(* Logix 5000 AddOnInstructionDefinition export Banner_IOL_Analog_Converter_Param_v4; software revision 33.00; part 2 of 2 *)
(* tags used below, declared in another part *)
   Converter : Banner_Analog_Converter_v4;
   Port_Data : Banner_IOL_Port_v4;
   Port : DINT;
   Type : DINT;   // 0 for S15C U/I models. 1 for R45C U/I models. 2 for R45C UU/II double analog models.
   Local_Control : DINT;
   Command_Being_Processed : BOOL;
   Index_Write_Inprocess : INT;
   Index_Write_Control : INT;
   Update_Archive : BOOL;
   Inprocess_Index : DINT;
   Index : DINT;
   Index2 : DINT;
   Index3 : DINT;
(* Banner_IOL_Analog_Converter_Param_v4, continued *)

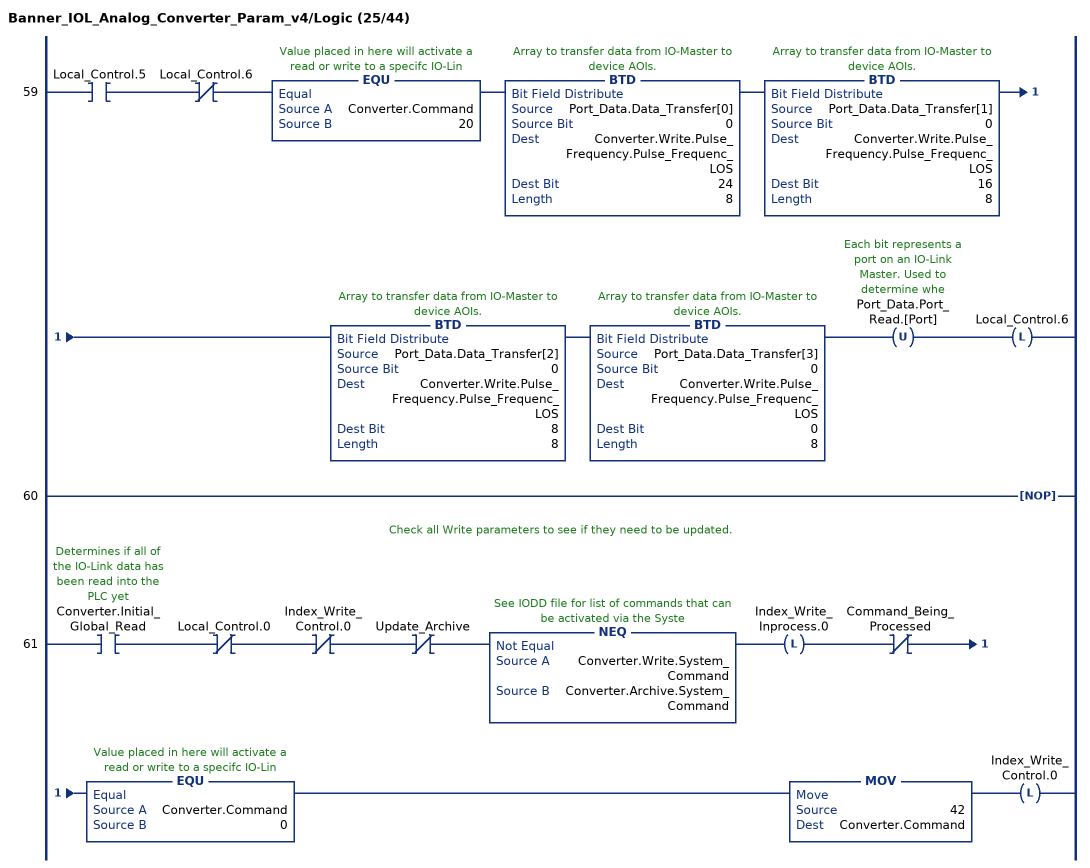
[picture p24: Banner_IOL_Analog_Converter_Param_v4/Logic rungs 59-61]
   59: XIC(Local_Control.5)XIO(Local_Control.6)EQU(Converter.Command,20)BTD(Port_Data.Data_Transfer[0],0,Converter.Write.Pulse_Frequency.Pulse_Frequenc_LOS,24,8)BTD(Port_Data.Data_Transfer[1],0,Converter.Write.Pulse_Frequency.Pulse_Frequenc_LOS,16,8)BTD(Port_Data.Data_Transfer[2],0,Converter.Write.Pulse_Frequency.Pulse_Frequenc_LOS,8,8)BTD(Port_Data.Data_Transfer[3],0,Converter.Write.Pulse_Frequency.Pulse_Frequenc_LOS,0,8)OTU(Port_Data.Port_Read.[Port])OTL(Local_Control.6);
   60: NOP();
   // Check all Write parameters to see if they need to be updated.
   61: XIC(Converter.Initial_Global_Read)XIO(Local_Control.0)XIO(Index_Write_Control.0)XIO(Update_Archive)NEQ(Converter.Write.System_Command,Converter.Archive.System_Command)OTL(Index_Write_Inprocess.0)XIO(Command_Being_Processed)EQU(Converter.Command,0)MOV(42,Converter.Command)OTL(Index_Write_Control.0);
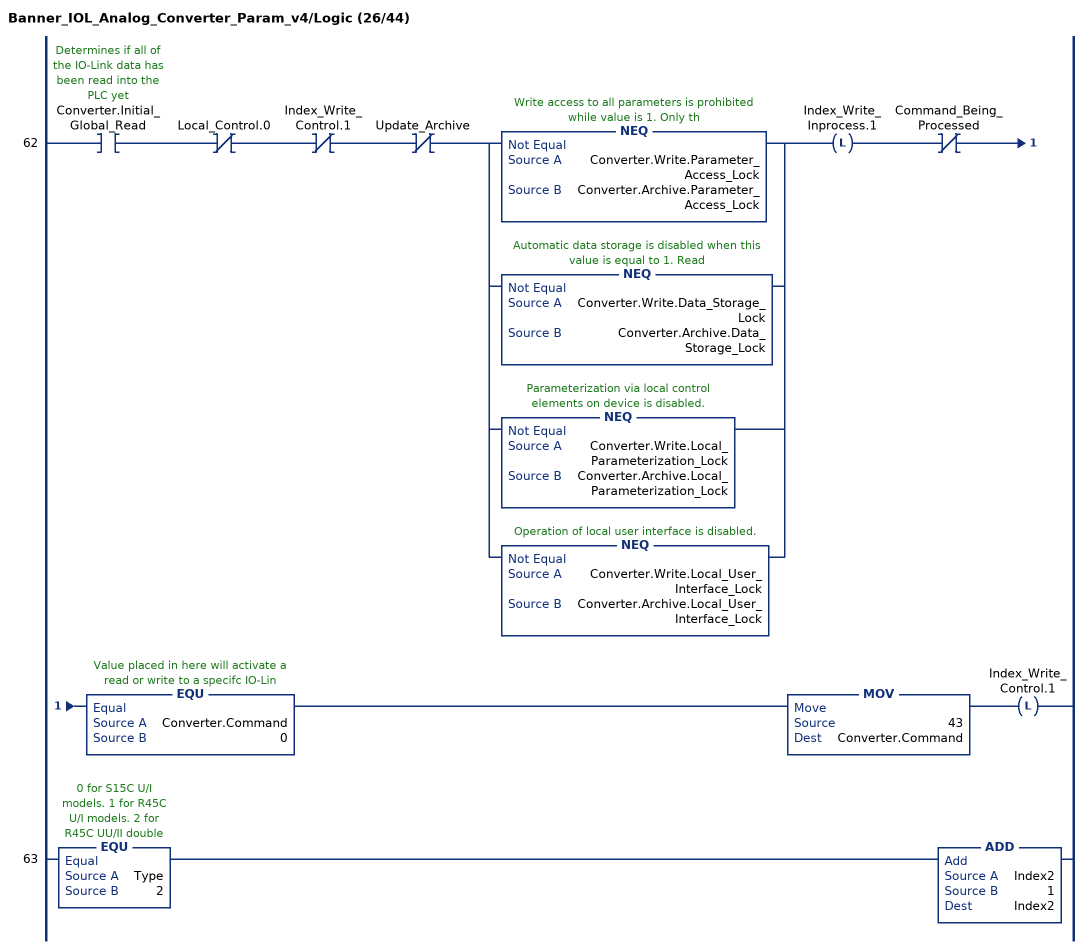
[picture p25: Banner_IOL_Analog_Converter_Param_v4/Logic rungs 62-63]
   62: XIC(Converter.Initial_Global_Read)XIO(Local_Control.0)XIO(Index_Write_Control.1)XIO(Update_Archive)[NEQ(Converter.Write.Parameter_Access_Lock,Converter.Archive.Parameter_Access_Lock) ,NEQ(Converter.Write.Data_Storage_Lock,Converter.Archive.Data_Storage_Lock) ,NEQ(Converter.Write.Local_Parameterization_Lock,Converter.Archive.Local_Parameterization_Lock) ,NEQ(Converter.Write.Local_User_Interface_Lock,Converter.Archive.Local_User_Interface_Lock) ]OTL(Index_Write_Inprocess.1)XIO(Command_Being_Processed)EQU(Converter.Command,0)MOV(43,Converter.Command)OTL(Index_Write_Control.1);
   63: EQU(Type,2)ADD(Index2,1,Index2);
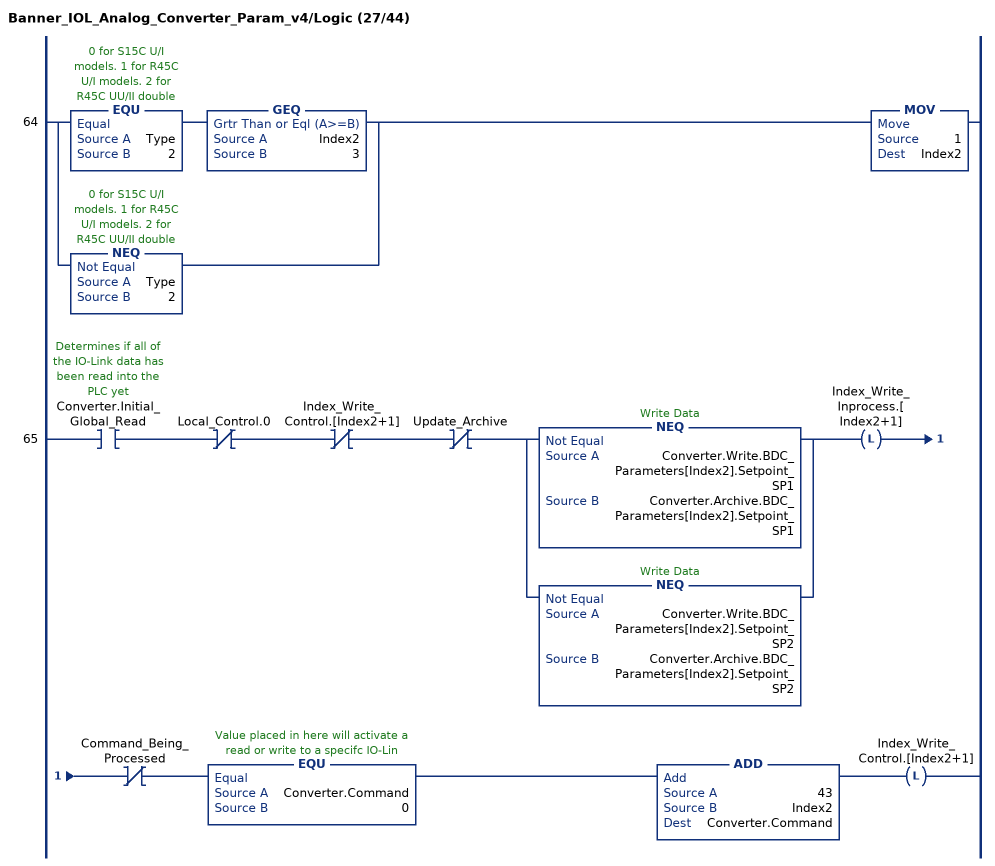
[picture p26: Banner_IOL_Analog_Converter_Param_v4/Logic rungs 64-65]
   64: [EQU(Type,2) GEQ(Index2,3) ,NEQ(Type,2) ]MOV(1,Index2);
   65: XIC(Converter.Initial_Global_Read)XIO(Local_Control.0)XIO(Index_Write_Control.[Index2+1])XIO(Update_Archive)[NEQ(Converter.Write.BDC_Parameters[Index2].Setpoint_SP1,Converter.Archive.BDC_Parameters[Index2].Setpoint_SP1) ,NEQ(Converter.Write.BDC_Parameters[Index2].Setpoint_SP2,Converter.Archive.BDC_Parameters[Index2].Setpoint_SP2) ]OTL(Index_Write_Inprocess.[Index2+1])XIO(Command_Being_Processed)EQU(Converter.Command,0)ADD(43,Index2,Converter.Command)OTL(Index_Write_Control.[Index2+1]);
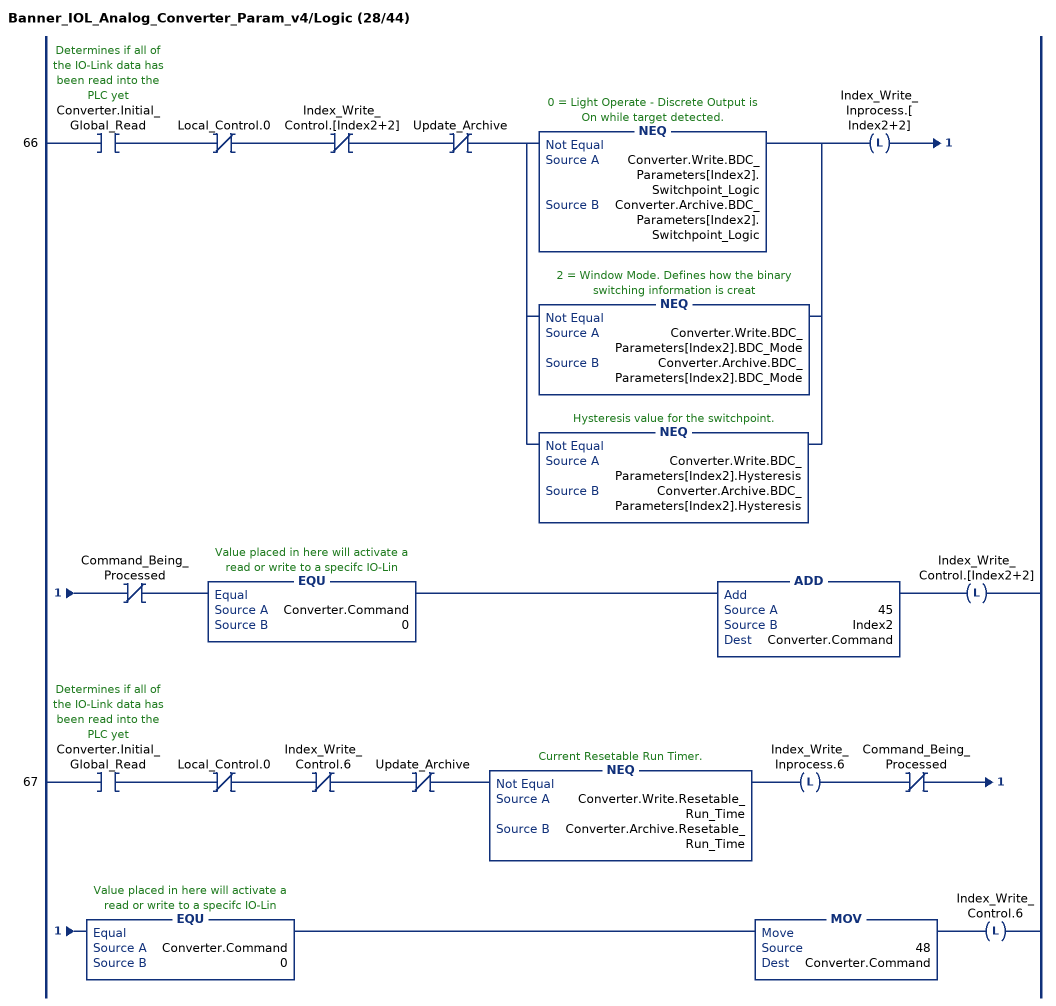
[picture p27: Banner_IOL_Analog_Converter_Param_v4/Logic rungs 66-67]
   66: XIC(Converter.Initial_Global_Read)XIO(Local_Control.0)XIO(Index_Write_Control.[Index2+2])XIO(Update_Archive)[NEQ(Converter.Write.BDC_Parameters[Index2].Switchpoint_Logic,Converter.Archive.BDC_Parameters[Index2].Switchpoint_Logic) ,NEQ(Converter.Write.BDC_Parameters[Index2].BDC_Mode,Converter.Archive.BDC_Parameters[Index2].BDC_Mode) ,NEQ(Converter.Write.BDC_Parameters[Index2].Hysteresis,Converter.Archive.BDC_Parameters[Index2].Hysteresis) ]OTL(Index_Write_Inprocess.[Index2+2])XIO(Command_Being_Processed)EQU(Converter.Command,0)ADD(45,Index2,Converter.Command)OTL(Index_Write_Control.[Index2+2]);
   67: XIC(Converter.Initial_Global_Read)XIO(Local_Control.0)XIO(Index_Write_Control.6)XIO(Update_Archive)NEQ(Converter.Write.Resetable_Run_Time,Converter.Archive.Resetable_Run_Time)OTL(Index_Write_Inprocess.6)XIO(Command_Being_Processed)EQU(Converter.Command,0)MOV(48,Converter.Command)OTL(Index_Write_Control.6);
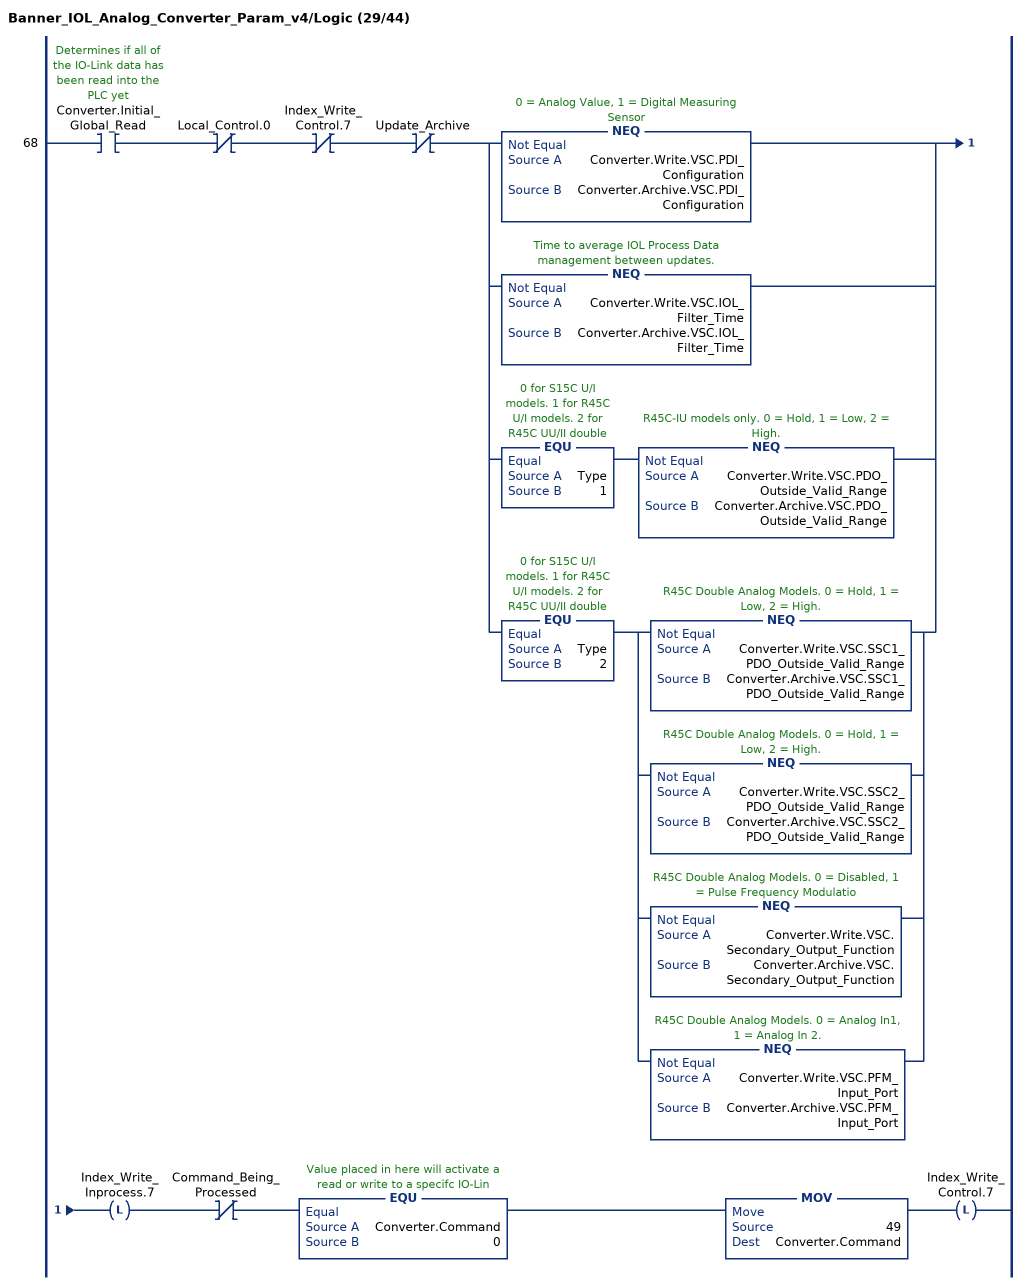
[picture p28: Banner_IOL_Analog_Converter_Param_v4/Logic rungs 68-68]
   68: XIC(Converter.Initial_Global_Read)XIO(Local_Control.0)XIO(Index_Write_Control.7)XIO(Update_Archive)[NEQ(Converter.Write.VSC.PDI_Configuration,Converter.Archive.VSC.PDI_Configuration) ,NEQ(Converter.Write.VSC.IOL_Filter_Time,Converter.Archive.VSC.IOL_Filter_Time) ,EQU(Type,1) NEQ(Converter.Write.VSC.PDO_Outside_Valid_Range,Converter.Archive.VSC.PDO_Outside_Valid_Range) ,EQU(Type,2) [NEQ(Converter.Write.VSC.SSC1_PDO_Outside_Valid_Range,Converter.Archive.VSC.SSC1_PDO_Outside_Valid_Range) ,NEQ(Converter.Write.VSC.SSC2_PDO_Outside_Valid_Range,Converter.Archive.VSC.SSC2_PDO_Outside_Valid_Range) ,NEQ(Converter.Write.VSC.Secondary_Output_Function,Converter.Archive.VSC.Secondary_Output_Function) ,NEQ(Converter.Write.VSC.PFM_Input_Port,Converter.Archive.VSC.PFM_Input_Port) ] ]OTL(Index_Write_Inprocess.7)XIO(Command_Being_Processed)EQU(Converter.Command,0)MOV(49,Converter.Command)OTL(Index_Write_Control.7);
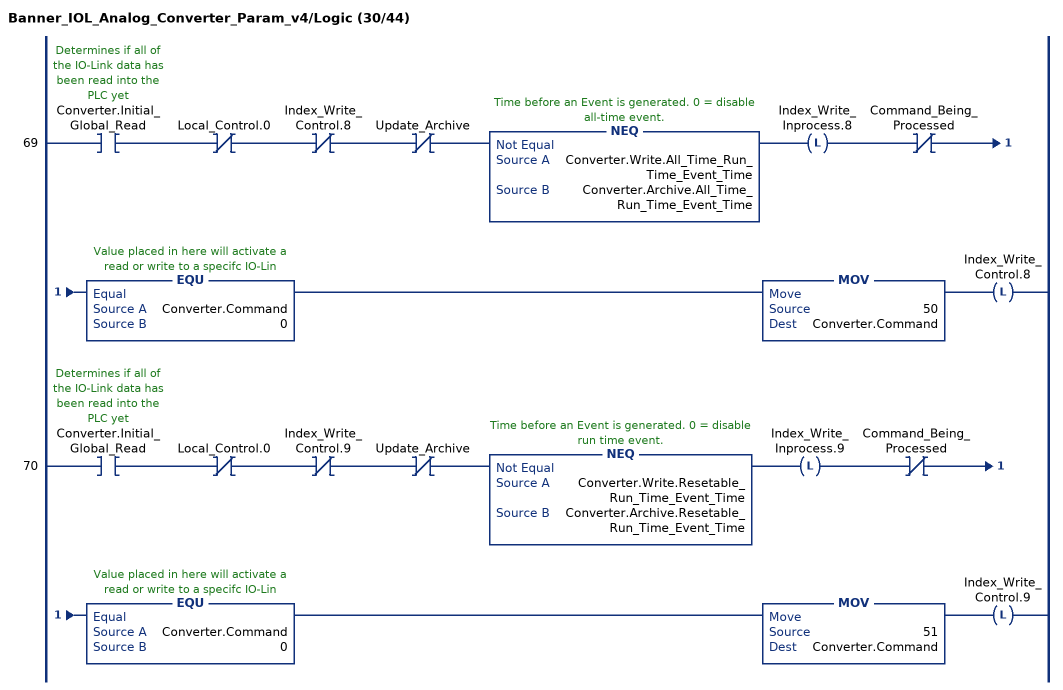
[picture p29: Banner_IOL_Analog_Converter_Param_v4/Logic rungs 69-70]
   69: XIC(Converter.Initial_Global_Read)XIO(Local_Control.0)XIO(Index_Write_Control.8)XIO(Update_Archive)NEQ(Converter.Write.All_Time_Run_Time_Event_Time,Converter.Archive.All_Time_Run_Time_Event_Time)OTL(Index_Write_Inprocess.8)XIO(Command_Being_Processed)EQU(Converter.Command,0)MOV(50,Converter.Command)OTL(Index_Write_Control.8);
   70: XIC(Converter.Initial_Global_Read)XIO(Local_Control.0)XIO(Index_Write_Control.9)XIO(Update_Archive)NEQ(Converter.Write.Resetable_Run_Time_Event_Time,Converter.Archive.Resetable_Run_Time_Event_Time)OTL(Index_Write_Inprocess.9)XIO(Command_Being_Processed)EQU(Converter.Command,0)MOV(51,Converter.Command)OTL(Index_Write_Control.9);
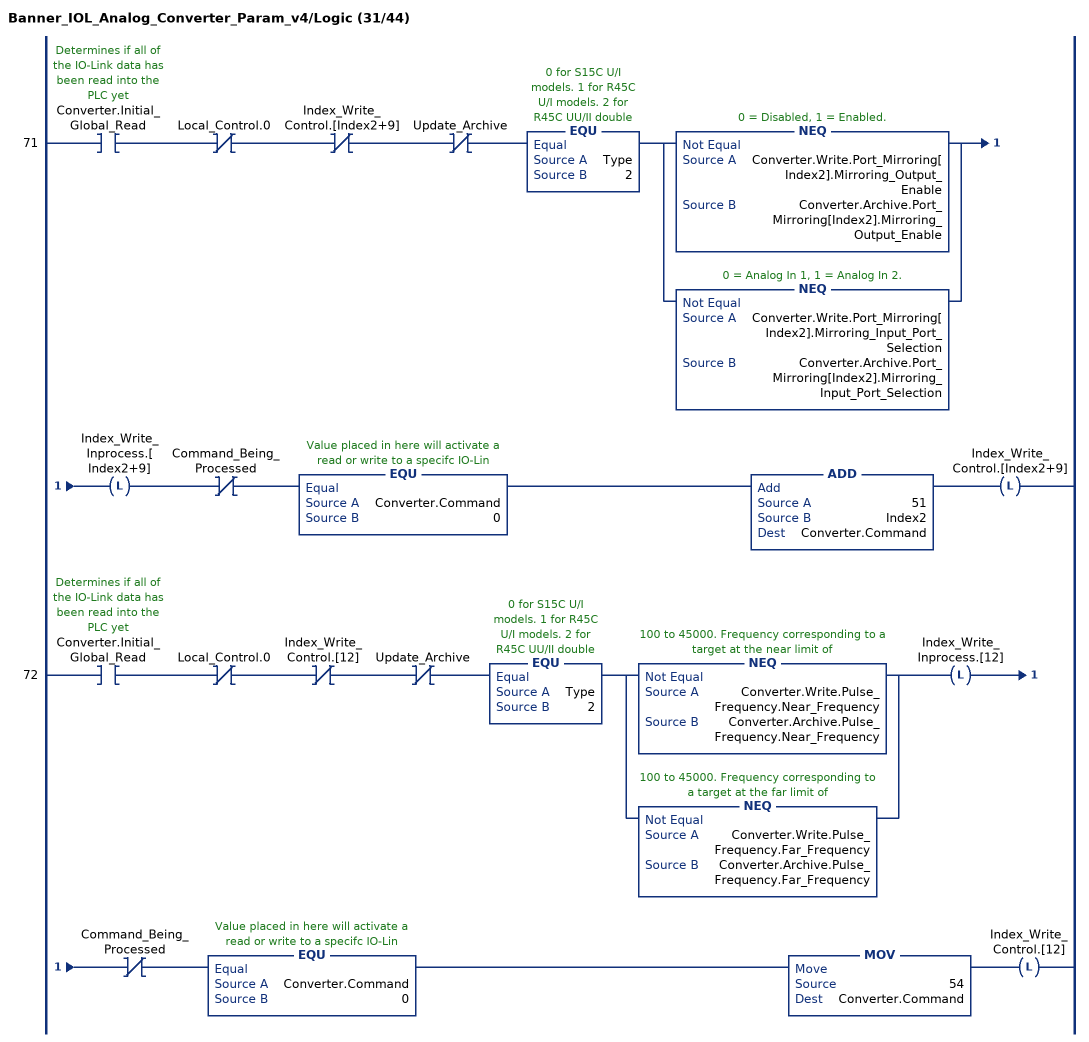
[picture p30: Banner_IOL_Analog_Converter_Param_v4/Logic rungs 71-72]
   71: XIC(Converter.Initial_Global_Read)XIO(Local_Control.0)XIO(Index_Write_Control.[Index2+9])XIO(Update_Archive)EQU(Type,2)[NEQ(Converter.Write.Port_Mirroring[Index2].Mirroring_Output_Enable,Converter.Archive.Port_Mirroring[Index2].Mirroring_Output_Enable) ,NEQ(Converter.Write.Port_Mirroring[Index2].Mirroring_Input_Port_Selection,Converter.Archive.Port_Mirroring[Index2].Mirroring_Input_Port_Selection) ]OTL(Index_Write_Inprocess.[Index2+9])XIO(Command_Being_Processed)EQU(Converter.Command,0)ADD(51,Index2,Converter.Command)OTL(Index_Write_Control.[Index2+9]);
   72: XIC(Converter.Initial_Global_Read)XIO(Local_Control.0)XIO(Index_Write_Control.[12])XIO(Update_Archive)EQU(Type,2)[NEQ(Converter.Write.Pulse_Frequency.Near_Frequency,Converter.Archive.Pulse_Frequency.Near_Frequency) ,NEQ(Converter.Write.Pulse_Frequency.Far_Frequency,Converter.Archive.Pulse_Frequency.Far_Frequency) ]OTL(Index_Write_Inprocess.[12])XIO(Command_Being_Processed)EQU(Converter.Command,0)MOV(54,Converter.Command)OTL(Index_Write_Control.[12]);
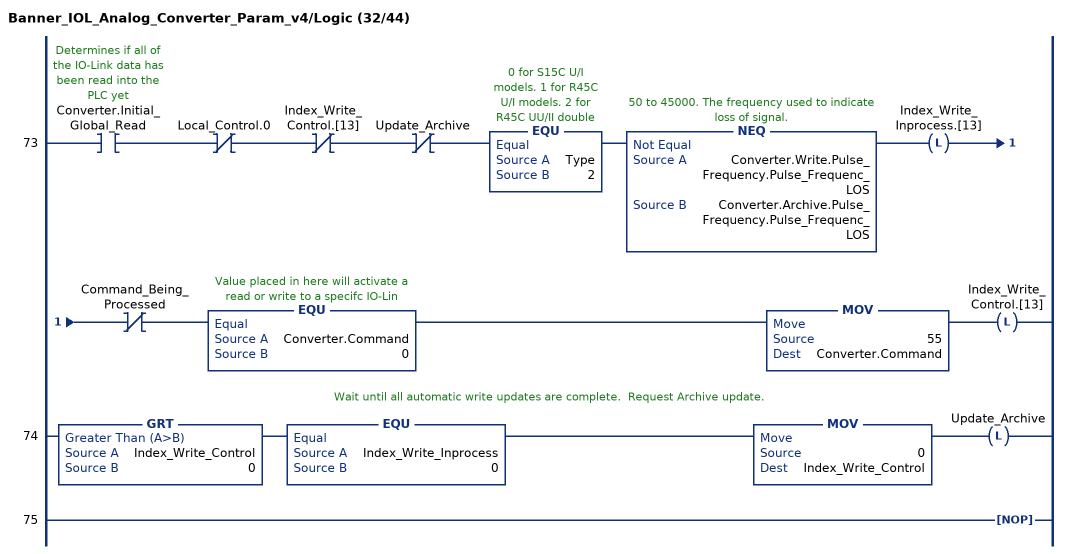
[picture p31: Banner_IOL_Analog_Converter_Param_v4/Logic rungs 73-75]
   73: XIC(Converter.Initial_Global_Read)XIO(Local_Control.0)XIO(Index_Write_Control.[13])XIO(Update_Archive)EQU(Type,2)NEQ(Converter.Write.Pulse_Frequency.Pulse_Frequenc_LOS,Converter.Archive.Pulse_Frequency.Pulse_Frequenc_LOS)OTL(Index_Write_Inprocess.[13])XIO(Command_Being_Processed)EQU(Converter.Command,0)MOV(55,Converter.Command)OTL(Index_Write_Control.[13]);
   // Wait until all automatic write updates are complete.  Request Archive update.
   74: GRT(Index_Write_Control,0)EQU(Index_Write_Inprocess,0)MOV(0,Index_Write_Control)OTL(Update_Archive);
   75: NOP();
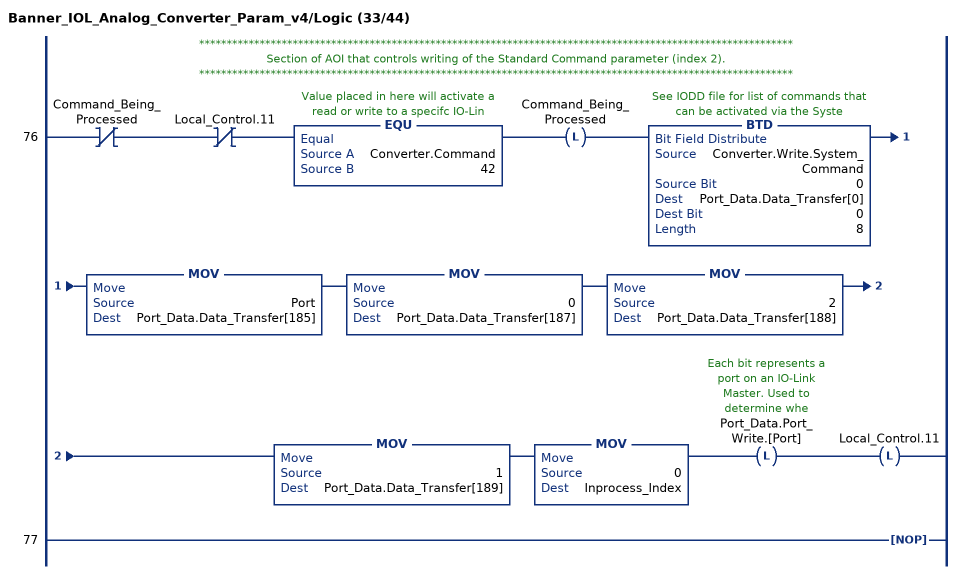
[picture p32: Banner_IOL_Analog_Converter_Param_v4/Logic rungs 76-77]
   // ************************************************************************************************************
   // Section of AOI that controls writing of the Standard Command parameter (index 2).
   // ************************************************************************************************************
   76: XIO(Command_Being_Processed)XIO(Local_Control.11)EQU(Converter.Command,42)OTL(Command_Being_Processed)BTD(Converter.Write.System_Command,0,Port_Data.Data_Transfer[0],0,8)MOV(Port,Port_Data.Data_Transfer[185])MOV(0,Port_Data.Data_Transfer[187])MOV(2,Port_Data.Data_Transfer[188])MOV(1,Port_Data.Data_Transfer[189])MOV(0,Inprocess_Index)OTL(Port_Data.Port_Write.[Port])OTL(Local_Control.11);
   77: NOP();
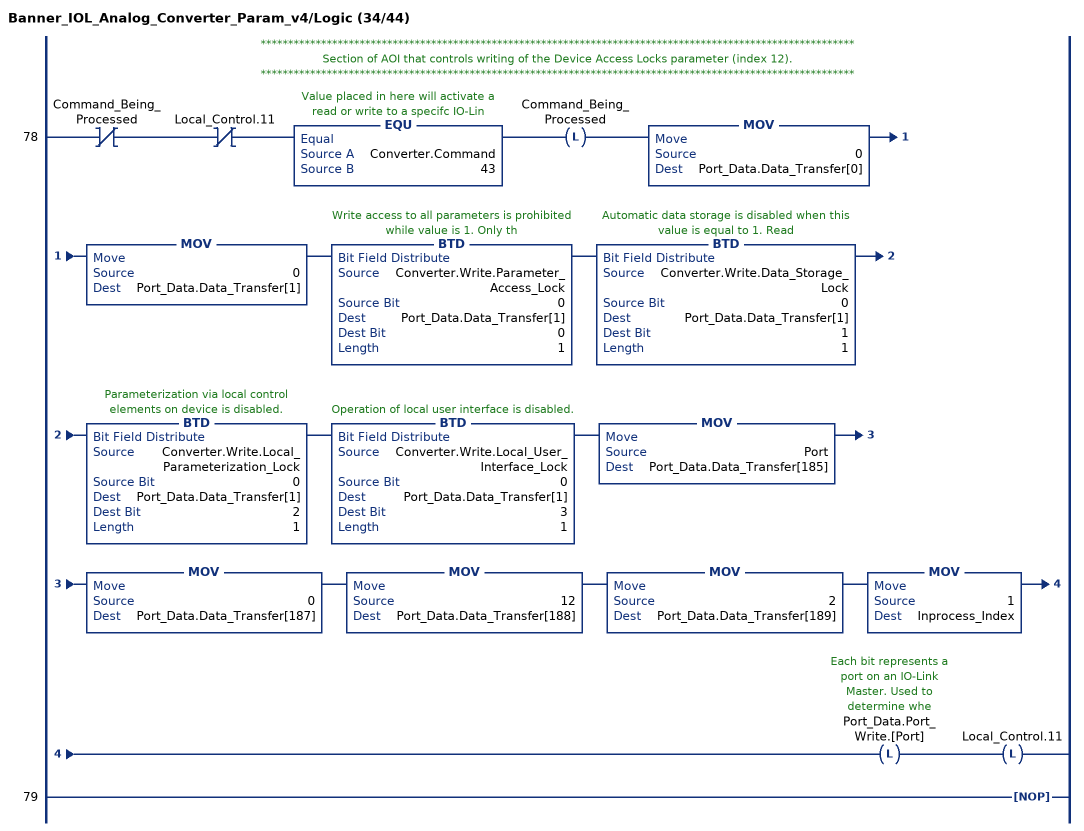
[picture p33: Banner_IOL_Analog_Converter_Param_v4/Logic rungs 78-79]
   // ************************************************************************************************************
   // Section of AOI that controls writing of the Device Access Locks parameter (index 12).
   // ************************************************************************************************************
   78: XIO(Command_Being_Processed)XIO(Local_Control.11)EQU(Converter.Command,43)OTL(Command_Being_Processed)MOV(0,Port_Data.Data_Transfer[0])MOV(0,Port_Data.Data_Transfer[1])BTD(Converter.Write.Parameter_Access_Lock,0,Port_Data.Data_Transfer[1],0,1)BTD(Converter.Write.Data_Storage_Lock,0,Port_Data.Data_Transfer[1],1,1)BTD(Converter.Write.Local_Parameterization_Lock,0,Port_Data.Data_Transfer[1],2,1)BTD(Converter.Write.Local_User_Interface_Lock,0,Port_Data.Data_Transfer[1],3,1)MOV(Port,Port_Data.Data_Transfer[185])MOV(0,Port_Data.Data_Transfer[187])MOV(12,Port_Data.Data_Transfer[188])MOV(2,Port_Data.Data_Transfer[189])MOV(1,Inprocess_Index)OTL(Port_Data.Port_Write.[Port])OTL(Local_Control.11);
   79: NOP();
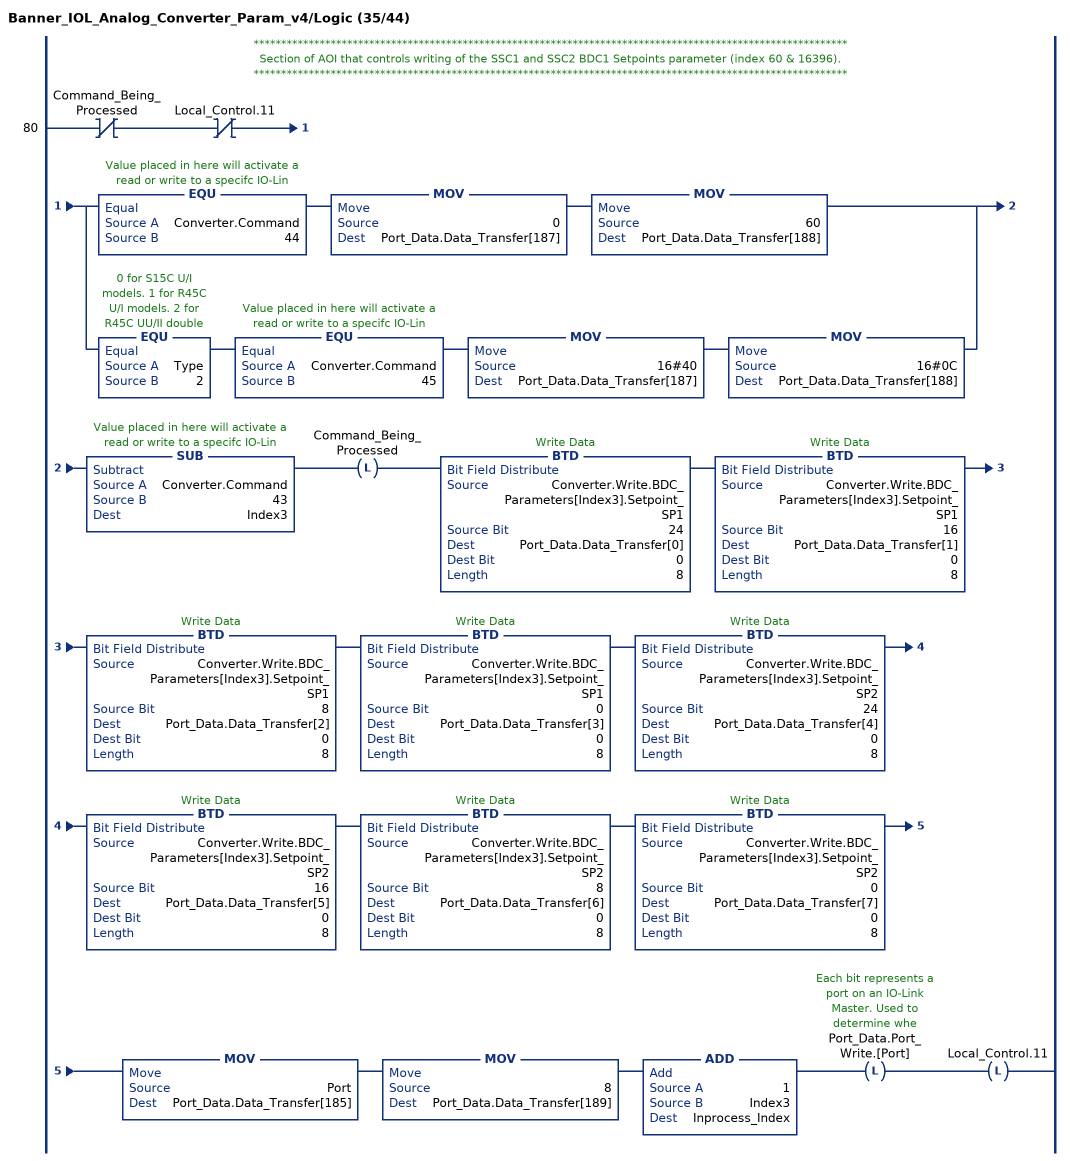
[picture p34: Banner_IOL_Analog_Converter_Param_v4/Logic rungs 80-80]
   // ************************************************************************************************************
   // Section of AOI that controls writing of the SSC1 and SSC2 BDC1 Setpoints parameter (index 60 & 16396).
   // ************************************************************************************************************
   80: XIO(Command_Being_Processed)XIO(Local_Control.11)[EQU(Converter.Command,44) MOV(0,Port_Data.Data_Transfer[187]) MOV(60,Port_Data.Data_Transfer[188]) ,EQU(Type,2) EQU(Converter.Command,45) MOV(16#40,Port_Data.Data_Transfer[187]) MOV(16#0C,Port_Data.Data_Transfer[188]) ]SUB(Converter.Command,43,Index3)OTL(Command_Being_Processed)BTD(Converter.Write.BDC_Parameters[Index3].Setpoint_SP1,24,Port_Data.Data_Transfer[0],0,8)BTD(Converter.Write.BDC_Parameters[Index3].Setpoint_SP1,16,Port_Data.Data_Transfer[1],0,8)BTD(Converter.Write.BDC_Parameters[Index3].Setpoint_SP1,8,Port_Data.Data_Transfer[2],0,8)BTD(Converter.Write.BDC_Parameters[Index3].Setpoint_SP1,0,Port_Data.Data_Transfer[3],0,8)BTD(Converter.Write.BDC_Parameters[Index3].Setpoint_SP2,24,Port_Data.Data_Transfer[4],0,8)BTD(Converter.Write.BDC_Parameters[Index3].Setpoint_SP2,16,Port_Data.Data_Transfer[5],0,8)BTD(Converter.Write.BDC_Parameters[Index3].Setpoint_SP2,8,Port_Data.Data_Transfer[6],0,8)BTD(Converter.Write.BDC_Parameters[Index3].Setpoint_SP2,0,Port_Data.Data_Transfer[7],0,8)MOV(Port,Port_Data.Data_Transfer[185])MOV(8,Port_Data.Data_Transfer[189])ADD(1,Index3,Inprocess_Index)OTL(Port_Data.Port_Write.[Port])OTL(Local_Control.11);
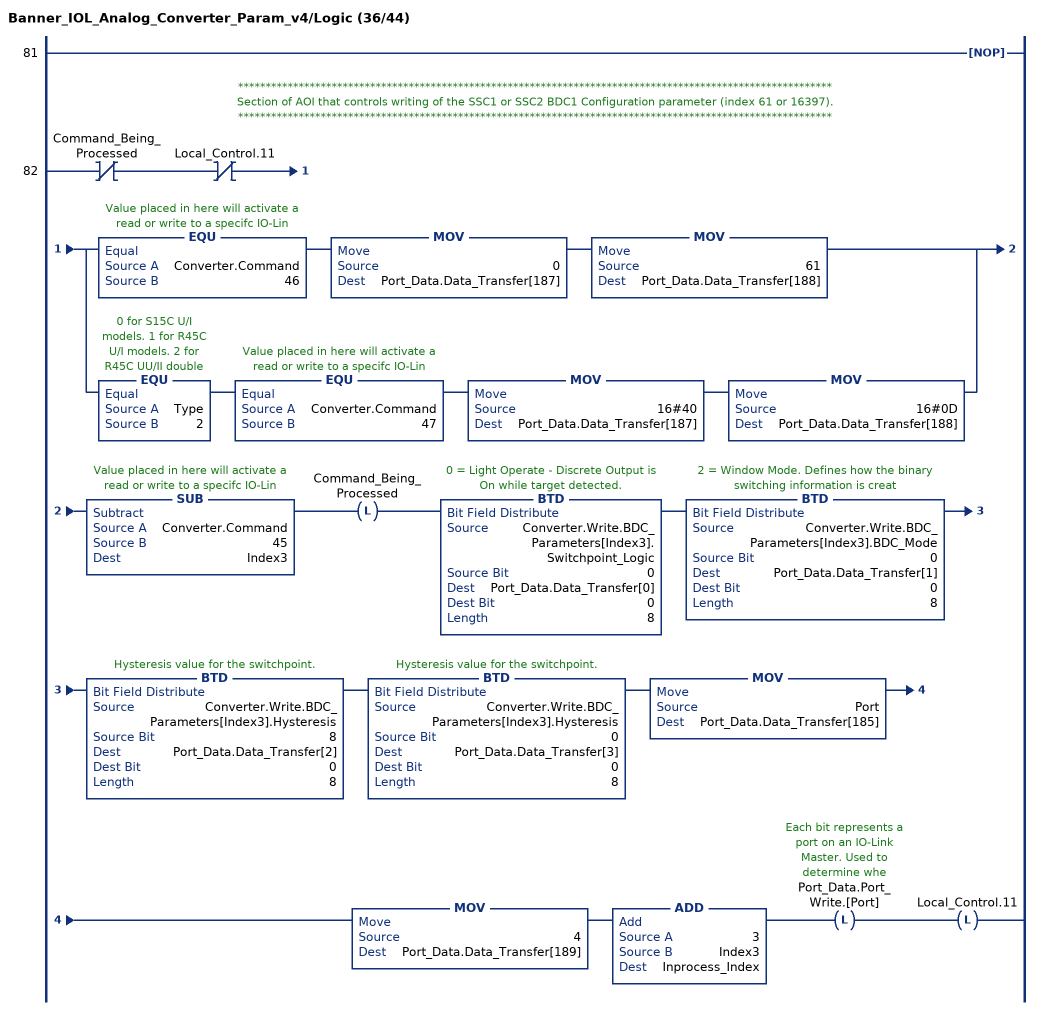
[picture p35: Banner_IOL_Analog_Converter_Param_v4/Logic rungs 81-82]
   81: NOP();
   // ************************************************************************************************************
   // Section of AOI that controls writing of the SSC1 or SSC2 BDC1 Configuration parameter (index 61 or 16397).
   // ************************************************************************************************************
   82: XIO(Command_Being_Processed)XIO(Local_Control.11)[EQU(Converter.Command,46) MOV(0,Port_Data.Data_Transfer[187]) MOV(61,Port_Data.Data_Transfer[188]) ,EQU(Type,2) EQU(Converter.Command,47) MOV(16#40,Port_Data.Data_Transfer[187]) MOV(16#0D,Port_Data.Data_Transfer[188]) ]SUB(Converter.Command,45,Index3)OTL(Command_Being_Processed)BTD(Converter.Write.BDC_Parameters[Index3].Switchpoint_Logic,0,Port_Data.Data_Transfer[0],0,8)BTD(Converter.Write.BDC_Parameters[Index3].BDC_Mode,0,Port_Data.Data_Transfer[1],0,8)BTD(Converter.Write.BDC_Parameters[Index3].Hysteresis,8,Port_Data.Data_Transfer[2],0,8)BTD(Converter.Write.BDC_Parameters[Index3].Hysteresis,0,Port_Data.Data_Transfer[3],0,8)MOV(Port,Port_Data.Data_Transfer[185])MOV(4,Port_Data.Data_Transfer[189])ADD(3,Index3,Inprocess_Index)OTL(Port_Data.Port_Write.[Port])OTL(Local_Control.11);
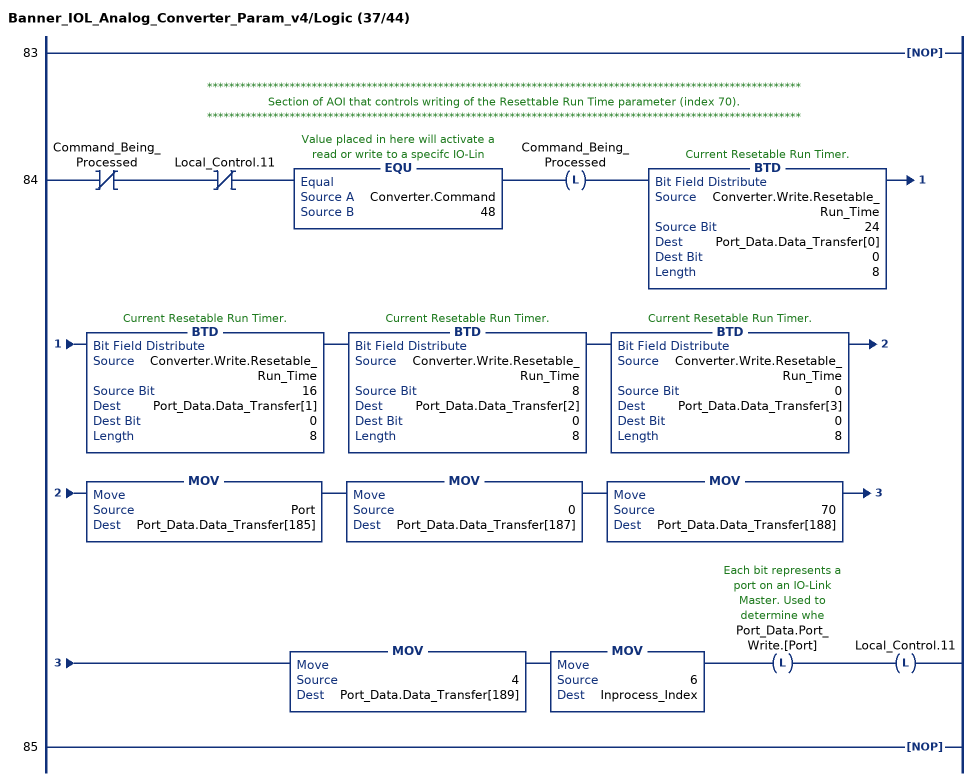
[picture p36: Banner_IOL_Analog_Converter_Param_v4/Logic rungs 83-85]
   83: NOP();
   // ************************************************************************************************************
   // Section of AOI that controls writing of the Resettable Run Time parameter (index 70).
   // ************************************************************************************************************
   84: XIO(Command_Being_Processed)XIO(Local_Control.11)EQU(Converter.Command,48)OTL(Command_Being_Processed)BTD(Converter.Write.Resetable_Run_Time,24,Port_Data.Data_Transfer[0],0,8)BTD(Converter.Write.Resetable_Run_Time,16,Port_Data.Data_Transfer[1],0,8)BTD(Converter.Write.Resetable_Run_Time,8,Port_Data.Data_Transfer[2],0,8)BTD(Converter.Write.Resetable_Run_Time,0,Port_Data.Data_Transfer[3],0,8)MOV(Port,Port_Data.Data_Transfer[185])MOV(0,Port_Data.Data_Transfer[187])MOV(70,Port_Data.Data_Transfer[188])MOV(4,Port_Data.Data_Transfer[189])MOV(6,Inprocess_Index)OTL(Port_Data.Port_Write.[Port])OTL(Local_Control.11);
   85: NOP();
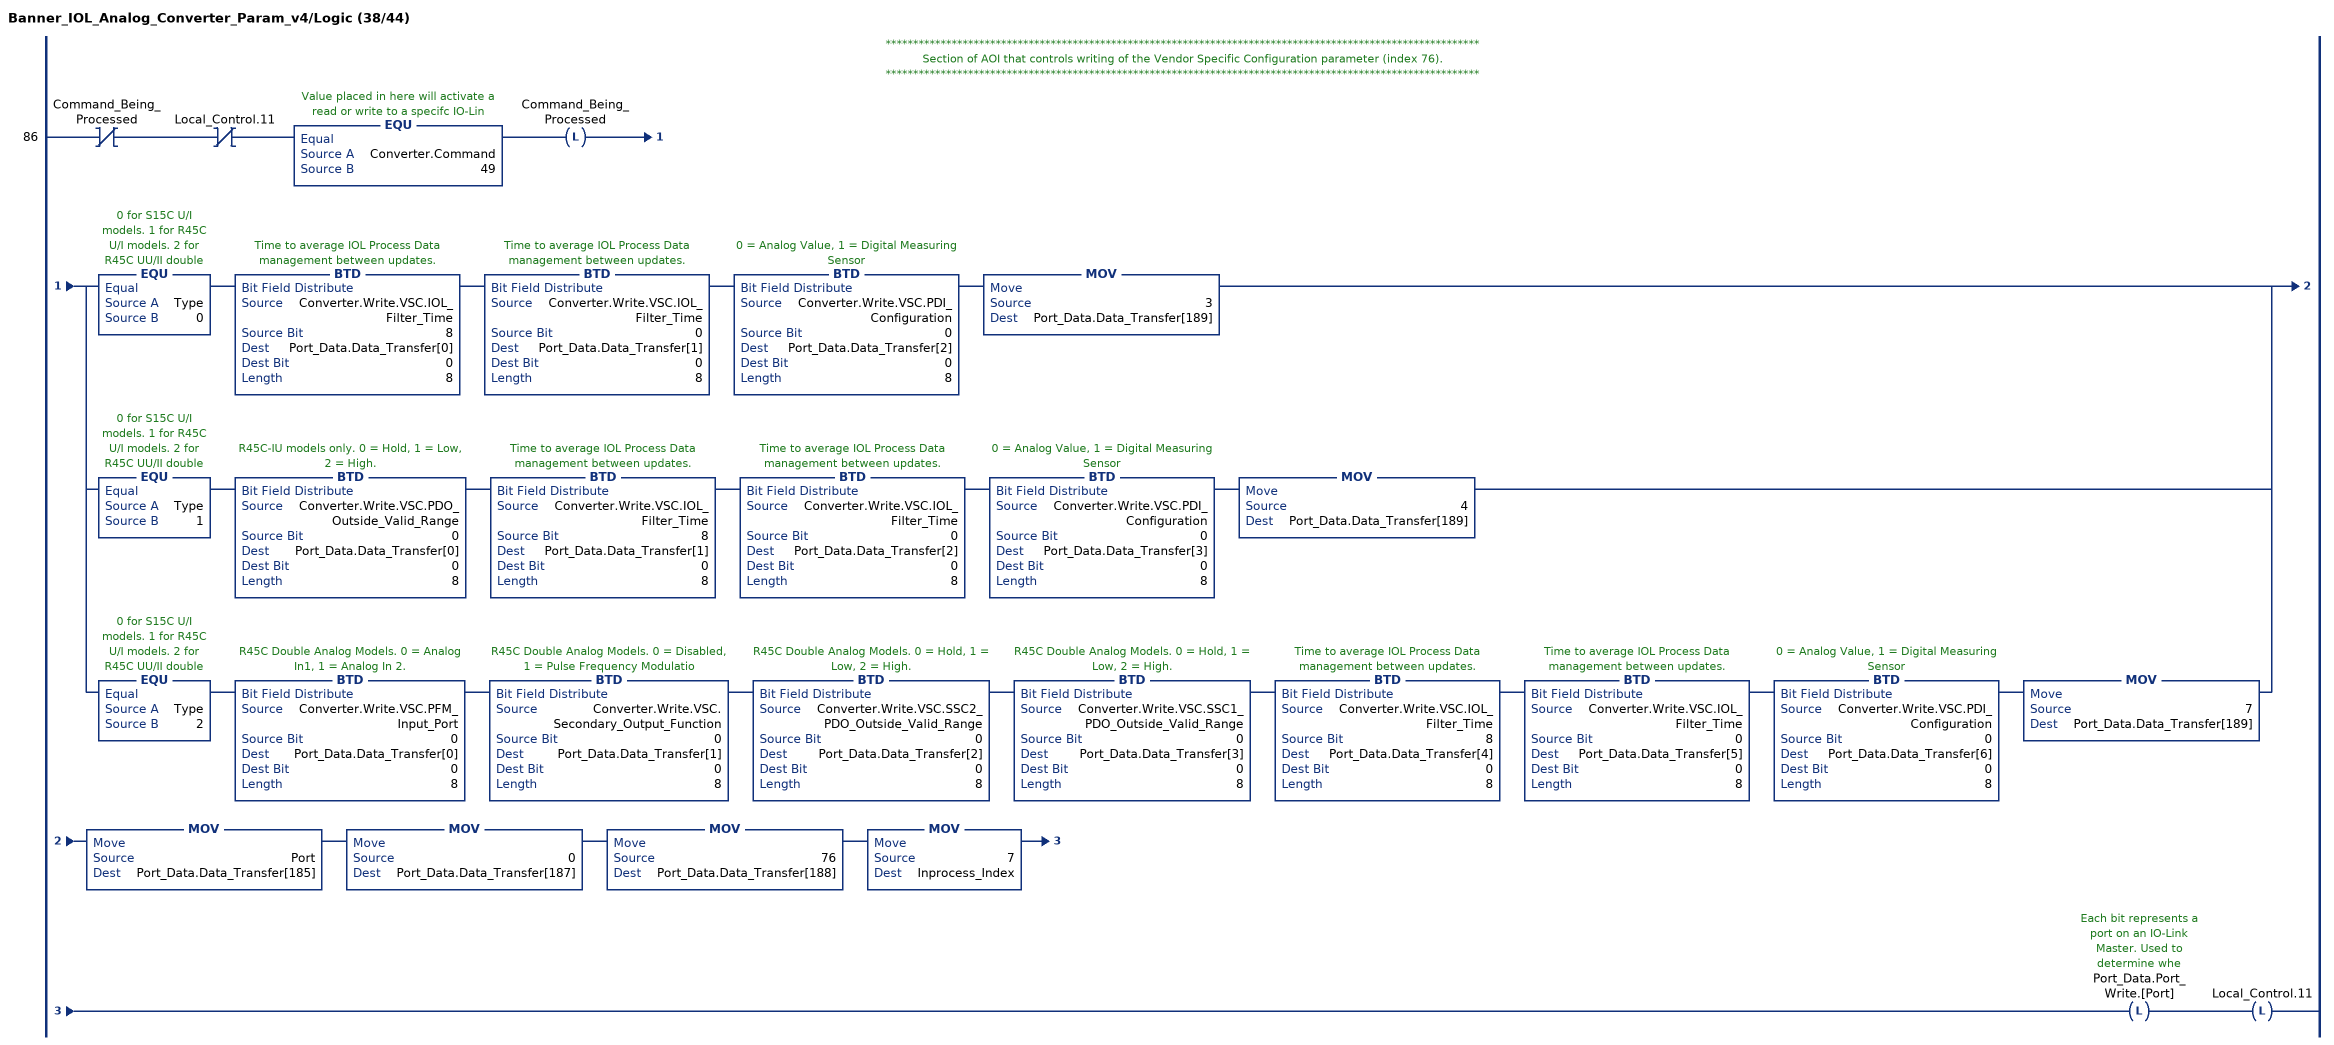
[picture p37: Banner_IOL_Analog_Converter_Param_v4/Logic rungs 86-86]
   // ************************************************************************************************************
   // Section of AOI that controls writing of the Vendor Specific Configuration parameter (index 76).
   // ************************************************************************************************************
   86: XIO(Command_Being_Processed)XIO(Local_Control.11)EQU(Converter.Command,49)OTL(Command_Being_Processed)[EQU(Type,0) BTD(Converter.Write.VSC.IOL_Filter_Time,8,Port_Data.Data_Transfer[0],0,8) BTD(Converter.Write.VSC.IOL_Filter_Time,0,Port_Data.Data_Transfer[1],0,8) BTD(Converter.Write.VSC.PDI_Configuration,0,Port_Data.Data_Transfer[2],0,8) MOV(3,Port_Data.Data_Transfer[189]) ,EQU(Type,1) BTD(Converter.Write.VSC.PDO_Outside_Valid_Range,0,Port_Data.Data_Transfer[0],0,8) BTD(Converter.Write.VSC.IOL_Filter_Time,8,Port_Data.Data_Transfer[1],0,8) BTD(Converter.Write.VSC.IOL_Filter_Time,0,Port_Data.Data_Transfer[2],0,8) BTD(Converter.Write.VSC.PDI_Configuration,0,Port_Data.Data_Transfer[3],0,8) MOV(4,Port_Data.Data_Transfer[189]) ,EQU(Type,2) BTD(Converter.Write.VSC.PFM_Input_Port,0,Port_Data.Data_Transfer[0],0,8) BTD(Converter.Write.VSC.Secondary_Output_Function,0,Port_Data.Data_Transfer[1],0,8) BTD(Converter.Write.VSC.SSC2_PDO_Outside_Valid_Range,0,Port_Data.Data_Transfer[2],0,8) BTD(Converter.Write.VSC.SSC1_PDO_Outside_Valid_Range,0,Port_Data.Data_Transfer[3],0,8) BTD(Converter.Write.VSC.IOL_Filter_Time,8,Port_Data.Data_Transfer[4],0,8) BTD(Converter.Write.VSC.IOL_Filter_Time,0,Port_Data.Data_Transfer[5],0,8) BTD(Converter.Write.VSC.PDI_Configuration,0,Port_Data.Data_Transfer[6],0,8) MOV(7,Port_Data.Data_Transfer[189]) ]MOV(Port,Port_Data.Data_Transfer[185])MOV(0,Port_Data.Data_Transfer[187])MOV(76,Port_Data.Data_Transfer[188])MOV(7,Inprocess_Index)OTL(Port_Data.Port_Write.[Port])OTL(Local_Control.11);
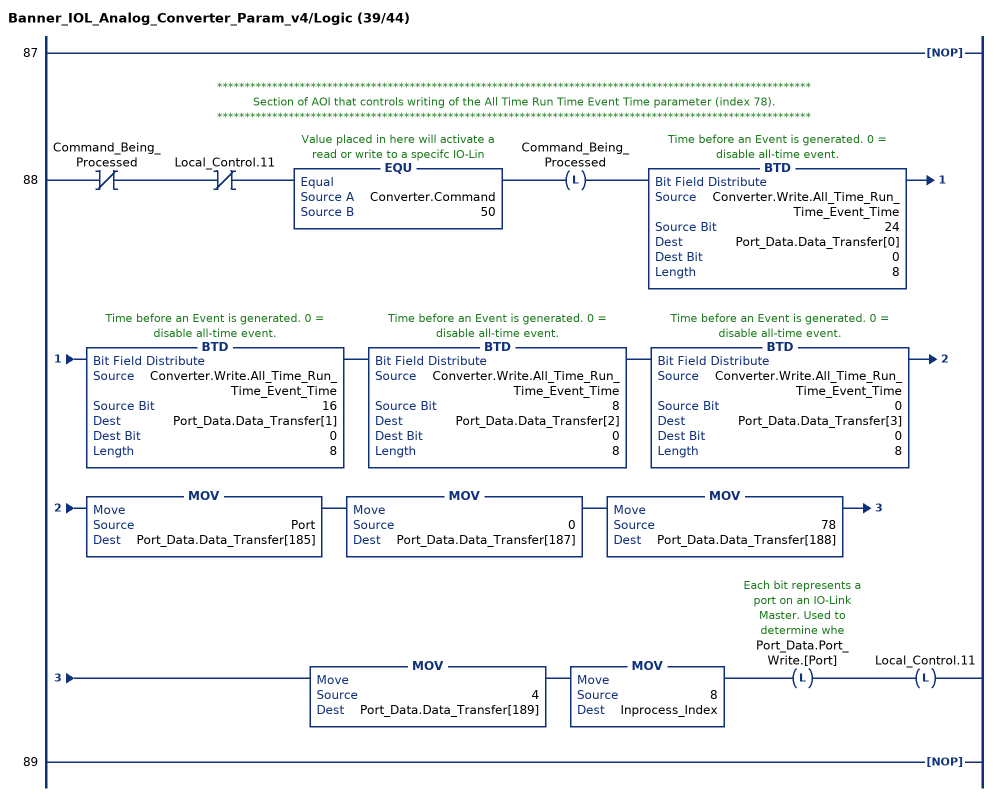
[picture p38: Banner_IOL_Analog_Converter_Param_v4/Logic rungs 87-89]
   87: NOP();
   // ************************************************************************************************************
   // Section of AOI that controls writing of the All Time Run Time Event Time parameter (index 78).
   // ************************************************************************************************************
   88: XIO(Command_Being_Processed)XIO(Local_Control.11)EQU(Converter.Command,50)OTL(Command_Being_Processed)BTD(Converter.Write.All_Time_Run_Time_Event_Time,24,Port_Data.Data_Transfer[0],0,8)BTD(Converter.Write.All_Time_Run_Time_Event_Time,16,Port_Data.Data_Transfer[1],0,8)BTD(Converter.Write.All_Time_Run_Time_Event_Time,8,Port_Data.Data_Transfer[2],0,8)BTD(Converter.Write.All_Time_Run_Time_Event_Time,0,Port_Data.Data_Transfer[3],0,8)MOV(Port,Port_Data.Data_Transfer[185])MOV(0,Port_Data.Data_Transfer[187])MOV(78,Port_Data.Data_Transfer[188])MOV(4,Port_Data.Data_Transfer[189])MOV(8,Inprocess_Index)OTL(Port_Data.Port_Write.[Port])OTL(Local_Control.11);
   89: NOP();
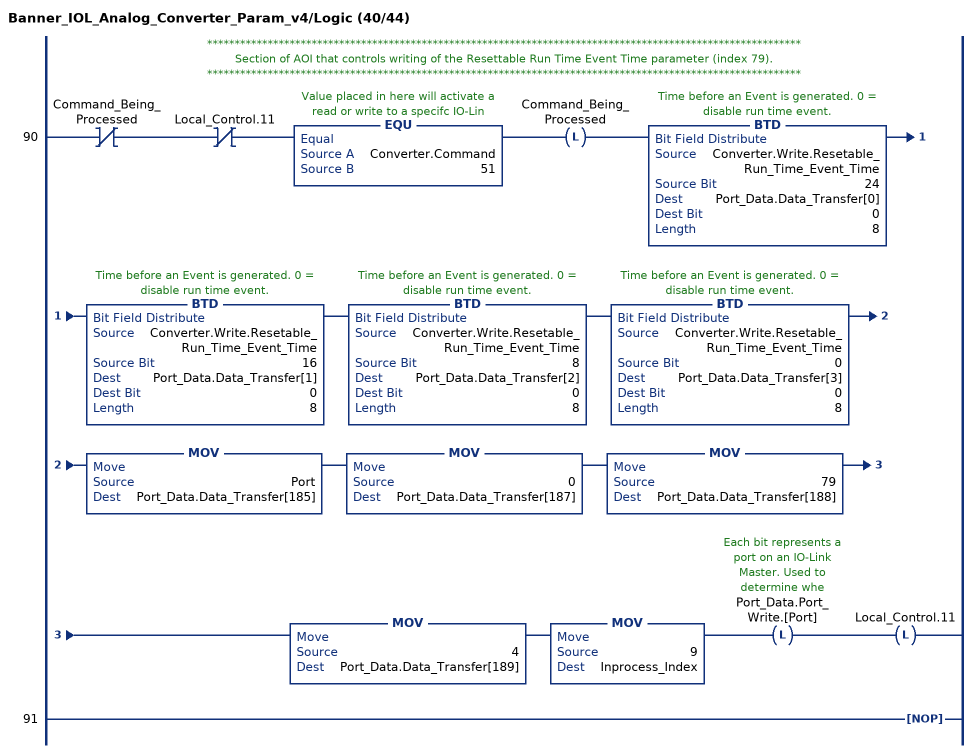
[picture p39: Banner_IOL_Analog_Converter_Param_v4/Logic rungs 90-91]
   // ************************************************************************************************************
   // Section of AOI that controls writing of the Resettable Run Time Event Time parameter (index 79).
   // ************************************************************************************************************
   90: XIO(Command_Being_Processed)XIO(Local_Control.11)EQU(Converter.Command,51)OTL(Command_Being_Processed)BTD(Converter.Write.Resetable_Run_Time_Event_Time,24,Port_Data.Data_Transfer[0],0,8)BTD(Converter.Write.Resetable_Run_Time_Event_Time,16,Port_Data.Data_Transfer[1],0,8)BTD(Converter.Write.Resetable_Run_Time_Event_Time,8,Port_Data.Data_Transfer[2],0,8)BTD(Converter.Write.Resetable_Run_Time_Event_Time,0,Port_Data.Data_Transfer[3],0,8)MOV(Port,Port_Data.Data_Transfer[185])MOV(0,Port_Data.Data_Transfer[187])MOV(79,Port_Data.Data_Transfer[188])MOV(4,Port_Data.Data_Transfer[189])MOV(9,Inprocess_Index)OTL(Port_Data.Port_Write.[Port])OTL(Local_Control.11);
   91: NOP();
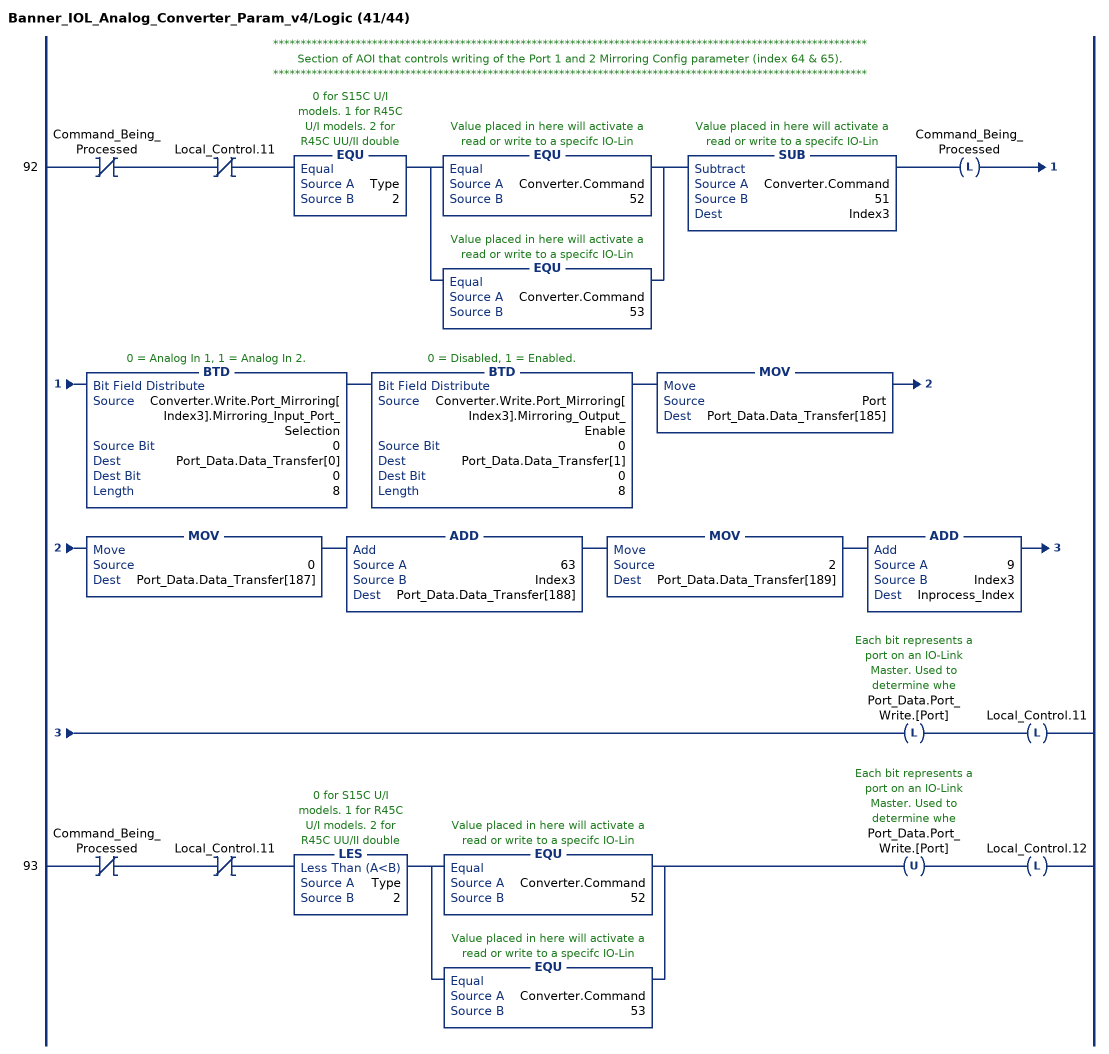
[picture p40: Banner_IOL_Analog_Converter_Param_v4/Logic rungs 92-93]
   // ************************************************************************************************************
   // Section of AOI that controls writing of the Port 1 and 2 Mirroring Config parameter (index 64 & 65).
   // ************************************************************************************************************
   92: XIO(Command_Being_Processed)XIO(Local_Control.11)EQU(Type,2)[EQU(Converter.Command,52) ,EQU(Converter.Command,53) ]SUB(Converter.Command,51,Index3)OTL(Command_Being_Processed)BTD(Converter.Write.Port_Mirroring[Index3].Mirroring_Input_Port_Selection,0,Port_Data.Data_Transfer[0],0,8)BTD(Converter.Write.Port_Mirroring[Index3].Mirroring_Output_Enable,0,Port_Data.Data_Transfer[1],0,8)MOV(Port,Port_Data.Data_Transfer[185])MOV(0,Port_Data.Data_Transfer[187])ADD(63,Index3,Port_Data.Data_Transfer[188])MOV(2,Port_Data.Data_Transfer[189])ADD(9,Index3,Inprocess_Index)OTL(Port_Data.Port_Write.[Port])OTL(Local_Control.11);
   93: XIO(Command_Being_Processed)XIO(Local_Control.11)LES(Type,2)[EQU(Converter.Command,52) ,EQU(Converter.Command,53) ]OTU(Port_Data.Port_Write.[Port])OTL(Local_Control.12);
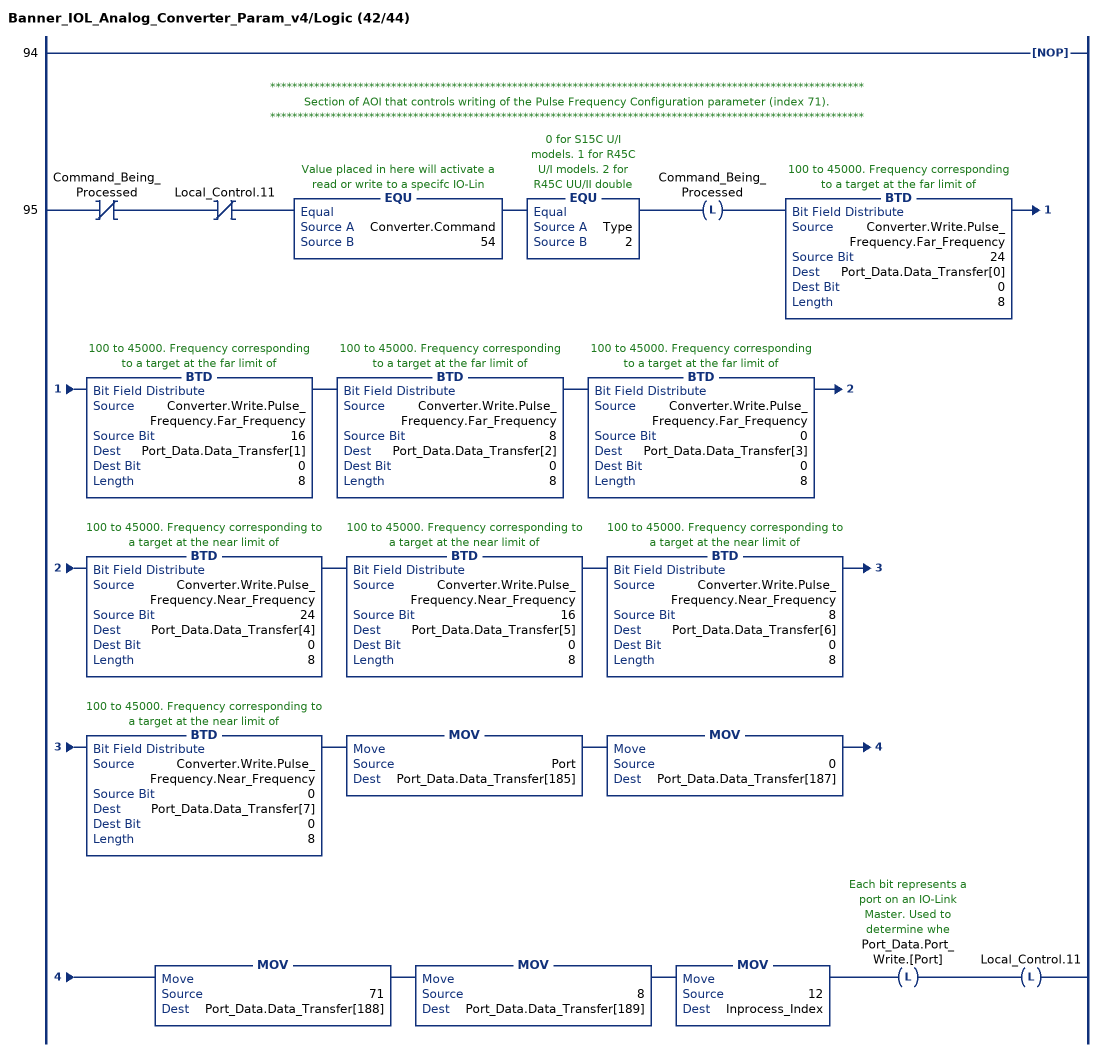
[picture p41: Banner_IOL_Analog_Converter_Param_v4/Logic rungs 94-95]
   94: NOP();
   // ************************************************************************************************************
   // Section of AOI that controls writing of the Pulse Frequency Configuration parameter (index 71).
   // ************************************************************************************************************
   95: XIO(Command_Being_Processed)XIO(Local_Control.11)EQU(Converter.Command,54)EQU(Type,2)OTL(Command_Being_Processed)BTD(Converter.Write.Pulse_Frequency.Far_Frequency,24,Port_Data.Data_Transfer[0],0,8)BTD(Converter.Write.Pulse_Frequency.Far_Frequency,16,Port_Data.Data_Transfer[1],0,8)BTD(Converter.Write.Pulse_Frequency.Far_Frequency,8,Port_Data.Data_Transfer[2],0,8)BTD(Converter.Write.Pulse_Frequency.Far_Frequency,0,Port_Data.Data_Transfer[3],0,8)BTD(Converter.Write.Pulse_Frequency.Near_Frequency,24,Port_Data.Data_Transfer[4],0,8)BTD(Converter.Write.Pulse_Frequency.Near_Frequency,16,Port_Data.Data_Transfer[5],0,8)BTD(Converter.Write.Pulse_Frequency.Near_Frequency,8,Port_Data.Data_Transfer[6],0,8)BTD(Converter.Write.Pulse_Frequency.Near_Frequency,0,Port_Data.Data_Transfer[7],0,8)MOV(Port,Port_Data.Data_Transfer[185])MOV(0,Port_Data.Data_Transfer[187])MOV(71,Port_Data.Data_Transfer[188])MOV(8,Port_Data.Data_Transfer[189])MOV(12,Inprocess_Index)OTL(Port_Data.Port_Write.[Port])OTL(Local_Control.11);
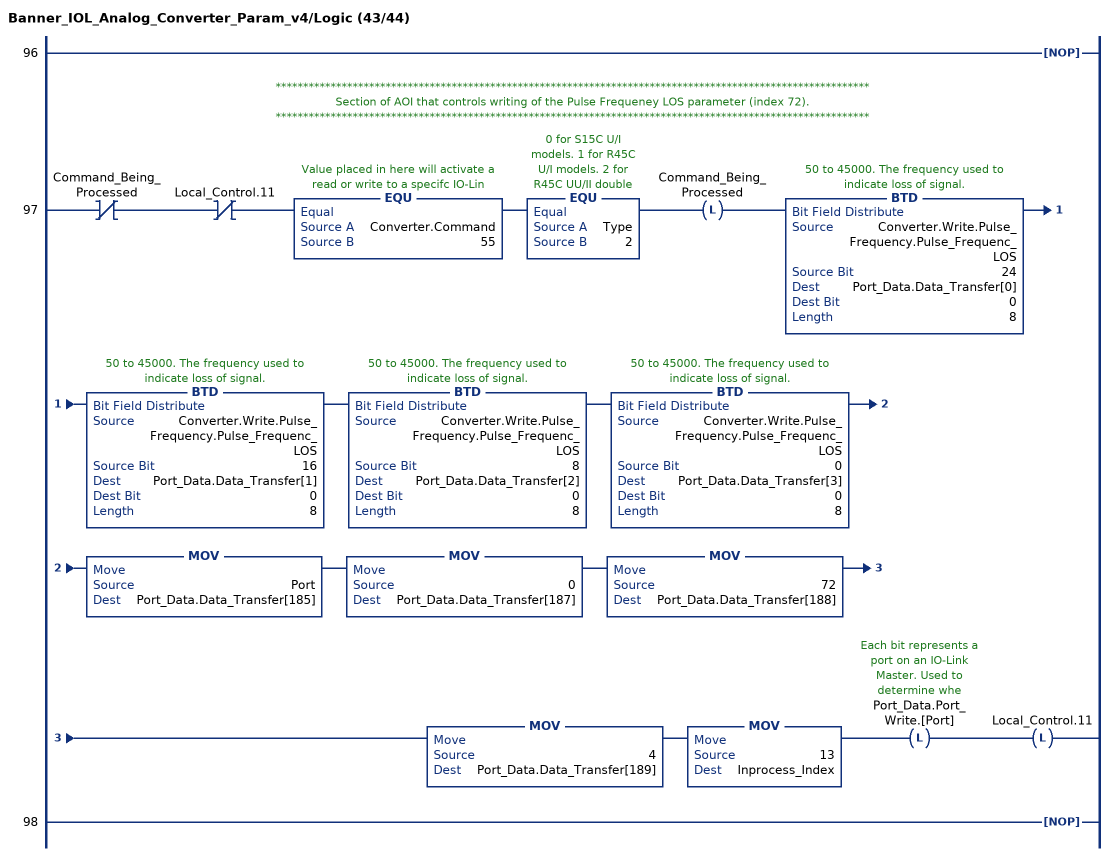
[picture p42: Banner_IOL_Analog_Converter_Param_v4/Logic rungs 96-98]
   96: NOP();
   // ************************************************************************************************************
   // Section of AOI that controls writing of the Pulse Frequeney LOS parameter (index 72).
   // ************************************************************************************************************
   97: XIO(Command_Being_Processed)XIO(Local_Control.11)EQU(Converter.Command,55)EQU(Type,2)OTL(Command_Being_Processed)BTD(Converter.Write.Pulse_Frequency.Pulse_Frequenc_LOS,24,Port_Data.Data_Transfer[0],0,8)BTD(Converter.Write.Pulse_Frequency.Pulse_Frequenc_LOS,16,Port_Data.Data_Transfer[1],0,8)BTD(Converter.Write.Pulse_Frequency.Pulse_Frequenc_LOS,8,Port_Data.Data_Transfer[2],0,8)BTD(Converter.Write.Pulse_Frequency.Pulse_Frequenc_LOS,0,Port_Data.Data_Transfer[3],0,8)MOV(Port,Port_Data.Data_Transfer[185])MOV(0,Port_Data.Data_Transfer[187])MOV(72,Port_Data.Data_Transfer[188])MOV(4,Port_Data.Data_Transfer[189])MOV(13,Inprocess_Index)OTL(Port_Data.Port_Write.[Port])OTL(Local_Control.11);
   98: NOP();
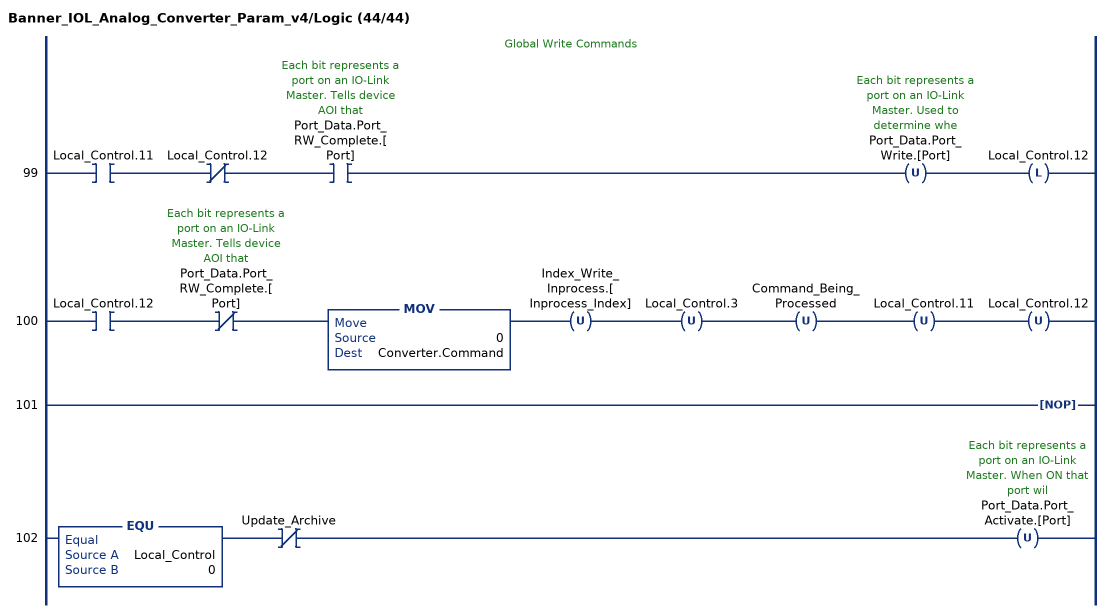
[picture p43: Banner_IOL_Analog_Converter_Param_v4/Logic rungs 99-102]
   // Global Write Commands
   99: XIC(Local_Control.11)XIO(Local_Control.12)XIC(Port_Data.Port_RW_Complete.[Port])OTU(Port_Data.Port_Write.[Port])OTL(Local_Control.12);
   100: XIC(Local_Control.12)XIO(Port_Data.Port_RW_Complete.[Port])MOV(0,Converter.Command)OTU(Index_Write_Inprocess.[Inprocess_Index])OTU(Local_Control.3)OTU(Command_Being_Processed)OTU(Local_Control.11)OTU(Local_Control.12);
   101: NOP();
   102: EQU(Local_Control,0)XIO(Update_Archive)OTU(Port_Data.Port_Activate.[Port]);
END_ROUTINE
END_ADD_ON_INSTRUCTION
